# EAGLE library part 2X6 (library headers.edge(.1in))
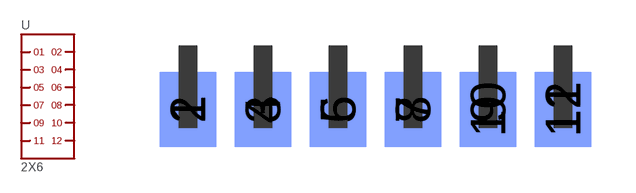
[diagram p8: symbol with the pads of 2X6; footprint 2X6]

Designator prefix -

## 2X6  [2X6]
1  1
2  2
3  3
4  4
5  5
6  6
7  7
8  8
9  9
10  10
11  11
12  12

## Footprint 2X6 (pad centres in mm)
smd 1.905 x 2.54: 1 0,-2.159; 3 2.54,-2.159; 5 5.08,-2.159; 7 7.62,-2.159; 9 10.16,-2.159; 11 12.7,-2.159
smd 1.905 x 2.54 bottom: 2 0,-2.159; 4 2.54,-2.159; 6 5.08,-2.159; 8 7.62,-2.159; 10 10.16,-2.159; 12 12.7,-2.159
